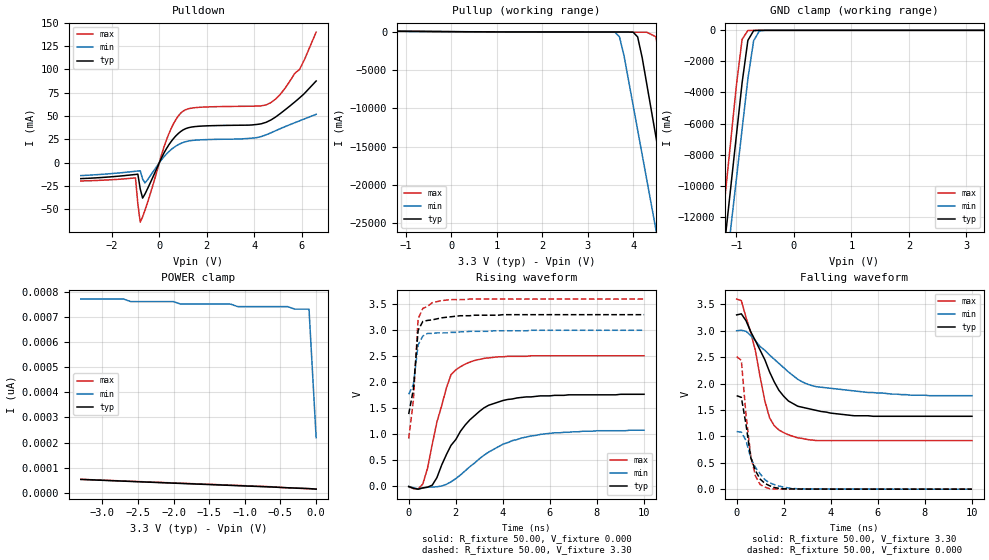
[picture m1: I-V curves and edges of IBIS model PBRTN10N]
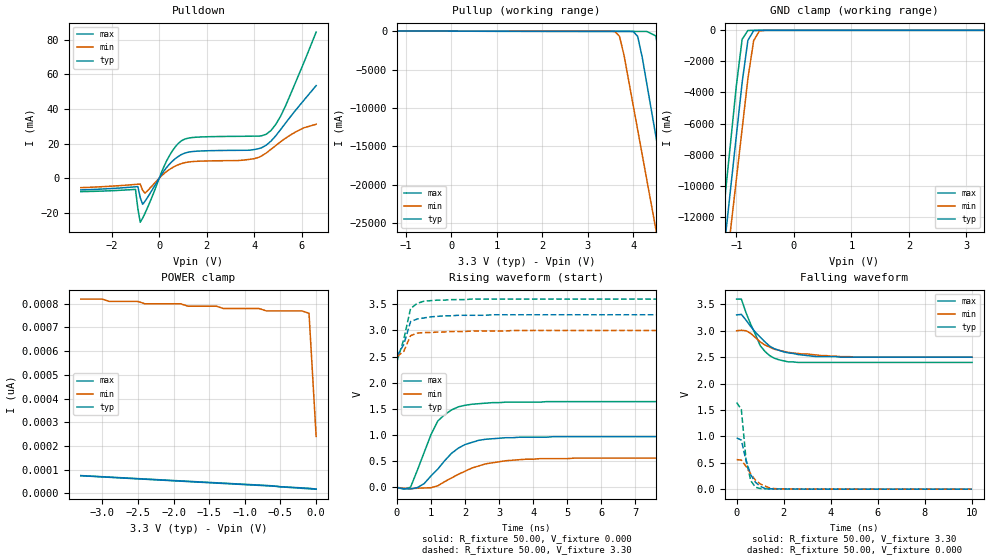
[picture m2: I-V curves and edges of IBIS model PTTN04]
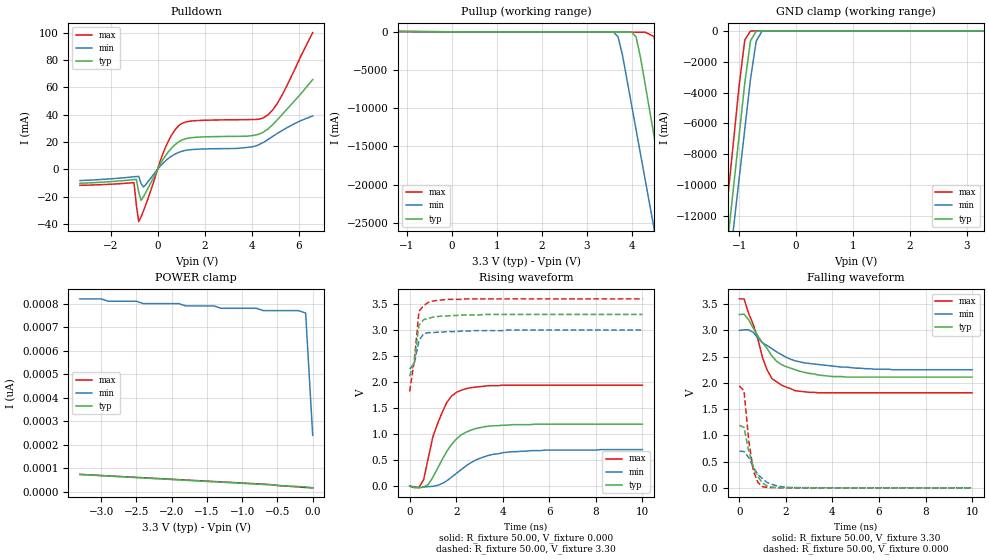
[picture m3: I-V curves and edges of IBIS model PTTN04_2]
| Integrated Devices Technolgy, Inc.
| IBIS MODEL OF 82v2048E
| PQFP_208
[Ibis Ver]   2.1
[File Name]   2048E_01.ibs
[File Rev]   2.0
[Date]   02/24/2002
[Source]   Integrated Devices Technolgy, Inc.
[Notes]   Spice type : spectre
[Disclaimer] Integrated Device Technology, Inc. ("IDT") hereby grants the
   user of this IBIS model a non-exclusive, nontransferable
   license to use this IBIS model under the following terms. The
   user is granted this license only to use the IBIS model and is
   not granted rights to sell, copy (except as needed to run the
   IBIS model), rent, lease or sub-license the IBIS model in
   whole or in part, or in modified form to anyone. The User may
   modify the IBIS model to suit its specific applications, but
   rights to derivative works and such modifications shall belong
   to IDT. This IBIS model is provided on an AS IS" basis and IDT
   makes absolutely no warranty with respect to the information
   contained herein. IDT DISCLAIMS AND CUSTOMER WAIVES ALL
   WARRANTIES, EXPRESS AND IMPLIED, INCLUDING WARRANTIES OF
   MERCHANTABILITY AND FITNESS FOR A PARTICULAR PURPOSE. THE
   ENTIRE RISK AS TO QUALITY AND PERFORMANCE IS WITH THE USER
   ACCORDINGLY, IN NO EVENT SHALL IDT BE LIABLE FOR ANY DIRECT OR
   INDIRECT DAMAGES, WHETHER IN CONTRACT OR TORT, INCLUDING ANY
   LOST PROFITS OR OTHER INCIDENTAL, CONSEQUENTIAL, EXEMPLARY, OR
   PUNITIVE DAMAGES ARISING OUT OF THE USE OR APPLICATION OF THE
   IBIS model. Further, IDT reserves the right to make changes
   without notice to any product herein to improve reliability,
   function, or design. IDT does not convey any license under
   patent rights or any other intellectual property rights,
   including those of third parties. IDT is not obligated to
   provide maintenance or support for the licensed IBIS model.
[Copyright]   Copyright 2002, Integrated Devices Technolgy, Inc. all rights
   reserved
|   Component 2048E_01 (PQFP_208)
[Component]   2048E_01
[Manufacturer]   Integrated Devices Technolgy, Inc.
[Package]
| variable   typ   min   max
R_pkg   178.7m   171.0m   186.4m
L_pkg   12.38nH   10.14nH   14.62nH
C_pkg   1.736pF   1.663pF   1.809pF
|   Pin List ( PQFP_208 )
[PIN]   signal_name   Model_name   R_pin   L_pin   C_pin
   1   LOS1   POTN04
   2   NC   NC
   3   LOS2   POTN04
   4   LOS3   POTN04
   5   LOS4   POTN04
   6   LOS5   POTN04
   7   LOS6   POTN04
   8   LOS7   POTN04
   9   LOS8   POTN04
   10   THZ   PITSN
   11   SCLKE   PITSN
   12   INT/MOT   PITSN
   13   IC   PITSN
   14   P/S   PITSN
   15   VDDD   POWER
   16   NC   NC
   17   MCLK   PITSN
   18   NC   NC
   19   GNDD   GND
   20   GNDIO   GND
   21   NC   NC
   22   VDDIO   POWER
   23   NC   NC
   24   D7   PBRTN10N
   25   D6   PBRTN10N
   26   D5   PBRTN10N
   27   D4   PBRTN10N
   28   D3   PBRTN10N
   29   D2   PBRTN10N
   30   D1   PBRTN10N
   31   D0   PBRTN10N
   32   NC   NC
   33   VDDIO   POWER
   34   TESTAPLL   POTN04
   35   GNDIO   GND
   36   NC   NC
   37   A7   PITSN
   38   A6   PITSN
   39   A5   PITSN
   40   A4   PITSN
   41   A3   PITSN
   42   A2   PITSN
   43   A1   PITSN
   44   A0   PITSN
   45   CS   PITSN
   46   SCLK   PITSN
   47   DS/RD   PITSN
   48   SDI/RW/WR   PITSN
   49   SDO   PTTN04_2
   50   INT   POTN04
   51   RST   PITSU
   52   NC   NC
   53   GPIO1   PBRTN10N
   54   GPIO0   PBRTN10N
   55   TESTSE   PITSN
   56   MCLKS   PITSN
   57   GNDA   GND
   58   TESTV   PAO
   59   REF   PAO
   60   VDDA   POWER
   61   VDDT   POWER
   62   VDDT   POWER
   63   TRING5   DRIVER
   64   TTIP5   DRIVER
   65   GNDT5   GND
   66   GNDT13   GND
   67   GNDR5   GND
   68   RRING5   PAI
   69   RTIP5   PAI
   70   VDDR5   POWER
   71   VDDR6   POWER
   72   RTIP6   PAI
   73   RRING6   PAI
   74   GNDR6   GND
   75   GNDT6   GND
   76   GNDT14   GND
   77   TTIP6   DRIVER
   78   TRING6   DRIVER
   79   VDDT   POWER
   80   VDDT   POWER
   81   VDDT   POWER
   82   VDDT   POWER
   83   TRING7   DRIVER
   84   TTIP7   DRIVER
   85   GNDT7   GND
   86   GNDT15   GND
   87   GNDR7   GND
   88   RRING7   PAI
   89   RTIP7   PAI
   90   VDDR7   POWER
   91   VDDR8   POWER
   92   RTIP8   PAI
   93   RRING8   PAI
   94   GNDR8   GND
   95   GNDT8   GND
   96   GNDT16   GND
   97   TTIP8   DRIVER
   98   TRING8   DRIVER
   99   VDDT   POWER
   100   VDDT   POWER
   101   NC   NC
   102   NC   NC
   103   VDDIO   POWER
   104   GNDIO   GND
   105   CV8/RDN8   PTTN04
   106   RD8/RDP8   PTTN04
   107   RCLK8   PTTN04_2
   108   TDN8   PITSN
   109   TD8/TDP8   PITSN
   110   TCLK8   PITSN
   111   CV7/RDN7   PTTN04
   112   RD7/RDP7   PTTN04
   113   RCLK7   PTTN04_2
   114   TDN7   PITSN
   115   TD7/TDP7   PITSN
   116   TCLK7   PITSN
   117   CV6/RDN6   PTTN04
   118   RD6/RDP6   PTTN04
   119   RCLK6   PTTN04_2
   120   TDN6   PITSN
   121   TD6/TDP6   PITSN
   122   TCLK6   PITSN
   123   CV5/RDN5   PTTN04
   124   RD5/RDP5   PTTN04
   125   RCLK5   PTTN04_2
   126   TDN5   PITSN
   127   TD5/TDP5   PITSN
   128   VDDIO   POWER
   129   TCLK5   PITSN
   130   GNDIO   GND
   131   GNDD   GND
   132   CV4/RDN4   PTTN04
   133   VDDD   POWER
   134   RD4/RDP4   PTTN04
   135   RCLK4   PTTN04_2
   136   TDN4   PITSN
   137   TD4/TDP4   PITSN
   138   TCLK4   PITSN
   139   CV3/RDN3   PTTN04
   140   RD3/RDP3   PTTN04
   141   RCLK3   PTTN04_2
   142   TDN3   PITSN
   143   TD3/TDP3   PITSN
   144   TCLK3   PITSN
   145   CV2/RDN2   PTTN04
   146   RD2/RDP2   PTTN04
   147   RCLK2   PTTN04_2
   148   TDN2   PITSN
   149   TD2/TDP2   PITSN
   150   TCLK2   PITSN
   151   CV1/RDN1   PTTN04
   152   RD1/RDP1   PTTN04
   153   RCLK1   PTTN04_2
   154   TDN1   PITSN
   155   TD1/TDP1   PITSN
   156   TCLK1   PITSN
   157   GNDIO   GND
   158   VDDIO   POWER
   159   NC   NC
   160   NC   NC
   161   VDDT   POWER
   162   VDDT   POWER
   163   TRING1   DRIVER
   164   TTIP1   DRIVER
   165   GNDT1   GND
   166   GNDT9   GND
   167   GNDR1   GND
   168   RRING1   PAI
   169   RTIP1   PAI
   170   VDDR1   POWER
   171   VDDR2   POWER
   172   RTIP2   PAI
   173   RRING2   PAI
   174   GNDR2   GND
   175   GNDT2   GND
   176   GNDT10   GND
   177   TTIP2   DRIVER
   178   TRING2   DRIVER
   179   VDDT   POWER
   180   VDDT   POWER
   181   VDDT   POWER
   182   VDDT   POWER
   183   TRING3   DRIVER
   184   TTIP3   DRIVER
   185   GNDT3   GND
   186   GNDT11   GND
   187   GNDR3   GND
   188   RRING3   PAI
   189   RTIP3   PAI
   190   VDDR3   POWER
   191   VDDR4   POWER
   192   RTIP4   PAI
   193   RRING4   PAI
   194   GNDR4   GND
   195   GNDT4   GND
   196   GNDT12   GND
   197   TTIP4   DRIVER
   198   TRING4   DRIVER
   199   VDDT   POWER
   200   VDDT   POWER
   201   VDDA   POWER
   202   NC   NC
   203   GNDA   GND
   204   TRST   PITSU
   205   TMS   PITSU
   206   TDI   PITSU
   207   TDO   PTTN04
   208   TCK   PITSN
| Models and submodels in the file (9): PBRTN10N (I/O), PTTN04 (3-state), PTTN04_2 (3-state), POTN04 (Output), PITSN (Input), PAI (Input), PITSU (Input), PAO (Input), DRIVER (3-state)
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|   Model PBRTN10N
[Model]   PBRTN10N
Model_type   I/O
Polarity   Non-Inverting
Enable   Active-Low
Vinl =   0.74V
Vinh =   2.10V
C_comp   3.50pF   4.00pF   3.20pF
[Temperature Range]   25.00   85.00   -40.00
[Voltage Range]   3.30V   3.00V   3.60V
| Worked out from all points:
|   slope of the pulldown table from 0 to 0.495 V, typ, clamps not added: 21.9 ohm
|   slope of the pullup table from 0 to 0.495 V, typ, clamps not added: 29.2 ohm
|   GND clamp passes 1 mA (typ) near -0.60 V on its own axis
|   rising waveform, R_fixture 50.00, V_fixture 0.000: 20-80 % time 1.59ns typ, 2.13ns min, 825ps max; typ from -0.002 V to 1.77 V
|   rising waveform, R_fixture 50.00, V_fixture 3.30: 20-80 % time 226ps typ, 225ps min, 235ps max; typ from 1.39 V to 3.3 V
|   falling waveform, R_fixture 50.00, V_fixture 3.30: 20-80 % time 1.32ns typ, 1.97ns min, 801ps max; typ from 3.3 V to 1.38 V
|   falling waveform, R_fixture 50.00, V_fixture 0.000: 20-80 % time 472ps typ, 702ps min, 384ps max; typ from 1.77 V to 0 V
[Pulldown]
| voltage   I(typ)   I(min)   I(max)
-3.3V     -16.95mA   -13.71mA   -19.45mA
-1V       -12.5mA    -9.06mA    -16.2mA
-900mV    -12.2mA    -8.75mA    -44.01mA
-800mV    -27.97mA   -8.57mA    -63.62mA
-700mV    -37.8mA    -17.39mA   -57.93mA
-600mV    -33.43mA   -21.55mA   -50.78mA
300mV     15.03mA    9.35mA     24.27mA
900mV     33.46mA    20.65mA    53.15mA
1.5V      38.77mA    24.19mA    59.03mA
4.7V      45.89mA    32.14mA    64.49mA
5.9V      69.46mA    44.93mA    100mA
6.6V      87.62mA    51.95mA    140mA
[Pullup]
| voltage   I(typ)   I(min)   I(max)
-3.3V     120mA      79.67mA    180mA
3.6V      -41.5mA    -64.51mA   -72.86mA
3.7V      -41.65mA   -690mA     -73.1mA
3.8V      -41.8mA    -3.15A     -73.33mA
4.1V      -690mA     -12.84A    -73.96mA
4.3V      -6.82A     -19.3A     -75.1mA
4.5V      -13.65A    -25.76A    -660mA
4.7V      -20.47A    -32.21A    -7.27A
4.9V      -27.29A    -38.67A    -14.54A
5.1V      -34.12A    -45.13A    -21.81A
5.3V      -40.94A    -51.59A    -29.07A
6.6V      -85.3A     -93.57A    -76.32A
[GND_clamp]
| voltage   I(typ)   I(min)   I(max)
-3.3V     -85.25A    -83.86A    -87.14A
-1.3V     -17.02A    -19.27A    -14.46A
-1.2V     -13.61A    -16.05A    -10.83A
-1.1V     -10.19A    -12.82A    -7.2A
-1V       -6.78A     -9.59A     -3.56A
-900mV    -3.37A     -6.36A     -580mA
-800mV    -650mA     -3.13A     -10.84mA
-700mV    -23.03mA   -670mA     -750uA
-600mV    -570uA     -40.72mA   -46.43uA
-400mV    -420nA     -76.92uA   -33.22nA
3.3V      15.23pA    730pA      12.85pA
[POWER_clamp]
| voltage   I(typ)   I(min)   I(max)
-3.3V     53.95pA    770pA      54.34pA
-2.7V     47.02pA    770pA      47.72pA
-2.6V     45.88pA    760pA      46.62pA
-2V       39.11pA    760pA      40.01pA
-1.9V     37.99pA    750pA      38.91pA
-1.2V     30.19pA    750pA      31.21pA
-1.1V     29.08pA    740pA      30.11pA
-400mV    20.85pA    740pA      20.54pA
-300mV    19.76pA    730pA      19.3pA
-100mV    17.59pA    730pA      17.04pA
0V        15.23pA    220pA      15.99pA
[Ramp]
| variable   typ   min   max
dV/dt_r   1.06/1.42n   0.65/2.13n   1.51/0.80n
dV/dt_f   1.15/1.32n   0.74/1.94n   1.61/0.81n
R_load = 50.00
[Rising Waveform]
R_fixture = 50.00
V_fixture = 0.000
V_fixture_min = 0.000
V_fixture_max = 0.000
| time   V(typ)   V(min)   V(max)
0s        -2.35mV    -1.01mV    -3.76mV
600ps     -28.68mV   -31.05mV   45.89mV
1ns       23.7mV     -11.09mV   810mV
1.6ns     610mV      39.29mV    1.89V
1.8ns     790mV      88.39mV    2.15V
2.2ns     1.06V      220mV      2.3V
3.2ns     1.51V      600mV      2.46V
4.2ns     1.67V      840mV      2.5V
6.2ns     1.75V      1.03V      2.51V
10ns      1.77V      1.08V      2.51V
[Rising Waveform]
R_fixture = 50.00
V_fixture = 3.30
V_fixture_min = 3.00
V_fixture_max = 3.60
| time   V(typ)   V(min)   V(max)
0s        1.39V      1.77V      920mV
200ps     1.87V      1.96V      1.66V
400ps     3V         2.72V      3.22V
600ps     3.17V      2.89V      3.42V
800ps     3.19V      2.94V      3.46V
1ns       3.2V       2.94V      3.53V
1.8ns     3.26V      2.96V      3.59V
2.8ns     3.29V      2.98V      3.6V
5.2ns     3.3V       3V         3.6V
10ns      3.3V       3V         3.6V
[Falling Waveform]
R_fixture = 50.00
V_fixture = 3.30
V_fixture_min = 3.00
V_fixture_max = 3.60
| time   V(typ)   V(min)   V(max)
0s        3.3V       3V         3.6V
200ps     3.32V      3.01V      3.57V
600ps     2.98V      2.91V      2.97V
800ps     2.81V      2.81V      2.62V
1.2ns     2.45V      2.63V      1.67V
1.4ns     2.22V      2.54V      1.35V
1.8ns     1.87V      2.38V      1.12V
2.6ns     1.57V      2.08V      970mV
3.4ns     1.49V      1.94V      920mV
10ns      1.38V      1.77V      920mV
[Falling Waveform]
R_fixture = 50.00
V_fixture = 0.000
V_fixture_min = 0.000
V_fixture_max = 0.000
| time   V(typ)   V(min)   V(max)
0s        1.77V      1.09V      2.51V
200ps     1.74V      1.08V      2.44V
400ps     1.22V      920mV      1.4V
600ps     600mV      590mV      630mV
800ps     350mV      410mV      250mV
1ns       190mV      290mV      86.54mV
1.4ns     65.04mV    120mV      8.44mV
1.8ns     15.51mV    59.38mV    3.46mV
2.4ns     4.08mV     13.27mV    1.63mV
10ns      1.37uV     -16.49uV   -7.85uV
|   Model PTTN04
[Model]   PTTN04
Model_type   3-state
Polarity   Non-Inverting
Enable   Active-Low
C_comp   3.50pF   4.00pF   3.50pF
[Temperature Range]   25.00   85.00   -40.00
[Voltage Range]   3.30V   3.00V   3.60V
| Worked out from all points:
|   slope of the pulldown table from 0 to 0.495 V, typ, clamps not added: 54.8 ohm
|   slope of the pullup table from 0 to 0.495 V, typ, clamps not added: 58.3 ohm
|   GND clamp passes 1 mA (typ) near -0.60 V on its own axis
|   rising waveform, R_fixture 50.00, V_fixture 0.000: 20-80 % time 911ps typ, 1.18ns min, 672ps max; typ from -0.001 V to 0.97 V
|   rising waveform, R_fixture 50.00, V_fixture 3.30: 20-80 % time 244ps typ, 200ps min, 267ps max; typ from 2.51 V to 3.3 V
|   falling waveform, R_fixture 50.00, V_fixture 3.30: 20-80 % time 1.1ns typ, 1.37ns min, 761ps max; typ from 3.3 V to 2.5 V
|   falling waveform, R_fixture 50.00, V_fixture 0.000: 20-80 % time 430ps typ, 596ps min, 274ps max; typ from 0.97 V to 0 V
[Pulldown]
| voltage   I(typ)   I(min)   I(max)
-3.3V     -6.78mA    -5.48mA    -7.78mA
-1V       -5mA       -3.62mA    -6.48mA
-900mV    -4.88mA    -3.5mA     -17.6mA
-800mV    -11.19mA   -3.43mA    -25.45mA
-700mV    -15.12mA   -6.95mA    -23.17mA
-600mV    -13.37mA   -8.62mA    -20.31mA
300mV     6.01mA     3.74mA     9.71mA
900mV     13.39mA    8.26mA     21.26mA
3.9V      16.33mA    11.07mA    24.26mA
4.7V      21.41mA    16.66mA    27.53mA
5.3V      31.61mA    22.97mA    41.38mA
6.6V      53.5mA     31.16mA    84.43mA
[Pullup]
| voltage   I(typ)   I(min)   I(max)
-3.3V     75.1mA     45.9mA     110mA
3.6V      -20.75mA   -52.61mA   -36.43mA
3.7V      -20.82mA   -680mA     -36.55mA
3.8V      -20.91mA   -3.14A     -36.66mA
4.1V      -670mA     -12.83A    -36.98mA
4.3V      -6.8A      -19.29A    -37.92mA
4.5V      -13.63A    -25.74A    -620mA
4.7V      -20.45A    -32.2A     -7.23A
4.9V      -27.27A    -38.66A    -14.5A
5.1V      -34.1A     -45.12A    -21.77A
5.3V      -40.92A    -51.58A    -29.04A
6.6V      -85.27A    -93.56A    -76.28A
[GND_clamp]
| voltage   I(typ)   I(min)   I(max)
-3.3V     -85.25A    -83.86A    -87.14A
-1.3V     -17.02A    -19.27A    -14.46A
-1.2V     -13.61A    -16.05A    -10.83A
-1.1V     -10.19A    -12.82A    -7.2A
-1V       -6.78A     -9.59A     -3.56A
-900mV    -3.37A     -6.36A     -580mA
-800mV    -650mA     -3.13A     -10.84mA
-700mV    -23.03mA   -670mA     -750uA
-600mV    -570uA     -40.72mA   -46.43uA
-400mV    -420nA     -76.92uA   -33.22nA
3.3V      17.37pA    770pA      12.87pA
[POWER_clamp]
| voltage   I(typ)   I(min)   I(max)
-3.3V     73.8pA     820pA      74.49pA
-2.5V     60.59pA    810pA      61.66pA
-2.4V     58.95pA    800pA      60.06pA
-1.9V     50.83pA    800pA      52.05pA
-1.8V     49.21pA    790pA      50.45pA
-1.4V     42.75pA    790pA      44.05pA
-1.3V     41.14pA    780pA      42.44pA
-800mV    33.09pA    780pA      34.44pA
-700mV    31.48pA    770pA      32.83pA
-200mV    22.54pA    770pA      20.69pA
-100mV    20.96pA    760pA      18.49pA
0V        17.27pA    240pA      17.07pA
[Ramp]
| variable   typ   min   max
dV/dt_r   0.58/0.86n   0.34/1.22n   0.98/0.61n
dV/dt_f   0.48/1.02n   0.30/1.52n   0.72/0.71n
R_load = 50.00
[Rising Waveform]
R_fixture = 50.00
V_fixture = 0.000
V_fixture_min = 0.000
V_fixture_max = 0.000
| time   V(typ)   V(min)   V(max)
0s        -1.28mV    -400uV     -2.34mV
200ps     -25mV      -16.44mV   -33.49mV
400ps     -28.55mV   -25.32mV   4.49mV
800ps     73.89mV    -10.55mV   670mV
1ns       220mV      -5.62mV    1.01V
1.2ns     350mV      31.07mV    1.27V
1.8ns     750mV      250mV      1.54V
2.4ns     900mV      410mV      1.6V
3.8ns     960mV      540mV      1.63V
10ns      970mV      560mV      1.64V
[Rising Waveform]
R_fixture = 50.00
V_fixture = 3.30
V_fixture_min = 3.00
V_fixture_max = 3.60
| time   V(typ)   V(min)   V(max)
0s        2.51V      2.5V       2.41V
200ps     2.73V      2.6V       2.83V
400ps     3.17V      2.9V       3.42V
600ps     3.22V      2.95V      3.52V
800ps     3.24V      2.96V      3.56V
1.4ns     3.28V      2.97V      3.58V
2.2ns     3.29V      2.99V      3.6V
2.8ns     3.3V       2.99V      3.6V
3.4ns     3.3V       3V         3.6V
10ns      3.3V       3V         3.6V
[Falling Waveform]
R_fixture = 50.00
V_fixture = 3.30
V_fixture_min = 3.00
V_fixture_max = 3.60
| time   V(typ)   V(min)   V(max)
0s        3.3V       3V         3.6V
200ps     3.31V      3.01V      3.6V
600ps     3.08V      2.95V      3.12V
1ns       2.88V      2.79V      2.72V
1.4ns     2.71V      2.69V      2.53V
1.8ns     2.63V      2.63V      2.45V
2.2ns     2.58V      2.59V      2.41V
3.4ns     2.51V      2.54V      2.4V
5ns       2.5V       2.5V       2.4V
10ns      2.5V       2.5V       2.4V
[Falling Waveform]
R_fixture = 50.00
V_fixture = 0.000
V_fixture_min = 0.000
V_fixture_max = 0.000
| time   V(typ)   V(min)   V(max)
0s        970mV      560mV      1.64V
200ps     930mV      550mV      1.51V
400ps     540mV      430mV      560mV
600ps     270mV      290mV      160mV
800ps     130mV      170mV      38.48mV
1ns       56mV       100mV      11.04mV
1.2ns     12.7mV     59.65mV    7.28mV
1.4ns     7.26mV     23.89mV    4.27mV
1.8ns     4.54mV     6.11mV     1.29mV
10ns      1.93uV     9.71uV     820nV
|   Model PTTN04_2
[Model]   PTTN04_2
Model_type   3-state
Polarity   Non-Inverting
Enable   Active-Low
C_comp   3.50pF   4.00pF   3.50pF
[Temperature Range]   25.00   85.00   -40.00
[Voltage Range]   3.30V   3.00V   3.60V
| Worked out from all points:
|   slope of the pulldown table from 0 to 0.495 V, typ, clamps not added: 36.6 ohm
|   slope of the pullup table from 0 to 0.495 V, typ, clamps not added: 46.6 ohm
|   GND clamp passes 1 mA (typ) near -0.60 V on its own axis
|   rising waveform, R_fixture 50.00, V_fixture 0.000: 20-80 % time 1.05ns typ, 1.49ns min, 812ps max; typ from -0.002 V to 1.19 V
|   rising waveform, R_fixture 50.00, V_fixture 3.30: 20-80 % time 233ps typ, 259ps min, 255ps max; typ from 2.11 V to 3.3 V
|   falling waveform, R_fixture 50.00, V_fixture 3.30: 20-80 % time 1.24ns typ, 1.8ns min, 816ps max; typ from 3.3 V to 2.11 V
|   falling waveform, R_fixture 50.00, V_fixture 0.000: 20-80 % time 481ps typ, 664ps min, 314ps max; typ from 1.19 V to 0 V
[Pulldown]
| voltage   I(typ)   I(min)   I(max)
-3.3V     -10.17mA   -8.22mA    -11.67mA
-1V       -7.5mA     -5.43mA    -9.72mA
-900mV    -7.32mA    -5.25mA    -26.41mA
-800mV    -16.78mA   -5.14mA    -38.17mA
-700mV    -22.68mA   -10.43mA   -34.76mA
-600mV    -20.06mA   -12.93mA   -30.47mA
300mV     9.02mA     5.61mA     14.56mA
800mV     18.81mA    11.62mA    30.08mA
1.3V      22.8mA     14.17mA    34.98mA
4.7V      29.57mA    21.83mA    39.85mA
5.3V      40.09mA    28.41mA    54.3mA
6.6V      65.68mA    39.04mA    100mA
[Pullup]
| voltage   I(typ)   I(min)   I(max)
-3.3V     86.33mA    53.19mA    130mA
3.6V      -25.94mA   -55.59mA   -45.54mA
3.7V      -26.03mA   -680mA     -45.69mA
3.8V      -26.13mA   -3.14A     -45.83mA
4.1V      -680mA     -12.83A    -46.23mA
4.3V      -6.81A     -19.29A    -47.22mA
4.5V      -13.63A    -25.75A    -630mA
4.7V      -20.46A    -32.21A    -7.24A
4.9V      -27.28A    -38.66A    -14.51A
5.1V      -34.1A     -45.12A    -21.78A
5.3V      -40.93A    -51.58A    -29.05A
6.6V      -85.28A    -93.56A    -76.29A
[GND_clamp]
| voltage   I(typ)   I(min)   I(max)
-3.3V     -85.25A    -83.86A    -87.14A
-1.3V     -17.02A    -19.27A    -14.46A
-1.2V     -13.61A    -16.05A    -10.83A
-1.1V     -10.19A    -12.82A    -7.2A
-1V       -6.78A     -9.59A     -3.56A
-900mV    -3.37A     -6.36A     -580mA
-800mV    -650mA     -3.13A     -10.84mA
-700mV    -23.03mA   -670mA     -750uA
-600mV    -570uA     -40.72mA   -46.43uA
-400mV    -420nA     -76.92uA   -33.22nA
3.3V      17.37pA    770pA      12.85pA
[POWER_clamp]
| voltage   I(typ)   I(min)   I(max)
-3.3V     73.8pA     820pA      74.44pA
-2.5V     60.58pA    810pA      61.62pA
-2.4V     58.95pA    800pA      60.02pA
-1.9V     50.82pA    800pA      52.01pA
-1.8V     49.21pA    790pA      50.41pA
-1.4V     42.75pA    790pA      44.01pA
-1.3V     41.13pA    780pA      42.41pA
-800mV    33.09pA    780pA      34.41pA
-700mV    31.48pA    770pA      32.8pA
-200mV    22.54pA    770pA      20.66pA
-100mV    20.96pA    760pA      18.46pA
0V        17.27pA    240pA      17.04pA
[Ramp]
| variable   typ   min   max
dV/dt_r   0.72/1.04n   0.42/1.49n   1.17/0.70n
dV/dt_f   0.71/1.19n   0.45/1.73n   1.07/0.81n
R_load = 50.00
[Rising Waveform]
R_fixture = 50.00
V_fixture = 0.000
V_fixture_min = 0.000
V_fixture_max = 0.000
| time   V(typ)   V(min)   V(max)
0s        -1.51mV    -530uV     -2.62mV
400ps     -35.79mV   -32.19mV   -25.03mV
600ps     -19.18mV   -19.59mV   120mV
1ns       170mV      -7.41mV    950mV
1.4ns     510mV      48.34mV    1.42V
1.8ns     800mV      170mV      1.73V
2.2ns     980mV      310mV      1.84V
3ns       1.12V      530mV      1.91V
4ns       1.17V      640mV      1.94V
10ns      1.19V      700mV      1.94V
[Rising Waveform]
R_fixture = 50.00
V_fixture = 3.30
V_fixture_min = 3.00
V_fixture_max = 3.60
| time   V(typ)   V(min)   V(max)
0s        2.11V      2.25V      1.82V
200ps     2.41V      2.36V      2.41V
400ps     3.09V      2.8V       3.36V
600ps     3.2V       2.93V      3.47V
800ps     3.22V      2.95V      3.53V
1ns       3.25V      2.95V      3.56V
1.6ns     3.27V      2.97V      3.59V
2.2ns     3.29V      2.98V      3.59V
3.2ns     3.3V       2.99V      3.6V
10ns      3.3V       3V         3.6V
[Falling Waveform]
R_fixture = 50.00
V_fixture = 3.30
V_fixture_min = 3.00
V_fixture_max = 3.60
| time   V(typ)   V(min)   V(max)
0s        3.3V       3V         3.6V
200ps     3.31V      3.01V      3.6V
600ps     3.04V      2.96V      3.11V
1ns       2.76V      2.76V      2.47V
1.2ns     2.65V      2.71V      2.24V
1.4ns     2.51V      2.65V      2.08V
2ns       2.31V      2.49V      1.92V
2.4ns     2.25V      2.42V      1.85V
4ns       2.12V      2.32V      1.81V
10ns      2.11V      2.25V      1.81V
[Falling Waveform]
R_fixture = 50.00
V_fixture = 0.000
V_fixture_min = 0.000
V_fixture_max = 0.000
| time   V(typ)   V(min)   V(max)
0s        1.19V      700mV      1.94V
200ps     1.15V      690mV      1.85V
400ps     710mV      580mV      910mV
600ps     400mV      390mV      320mV
800ps     210mV      250mV      99.86mV
1ns       88.8mV     170mV      21.99mV
1.2ns     33.22mV    99.38mV    7.33mV
1.4ns     12.02mV    66.22mV    5.32mV
2.2ns     3.35mV     5.86mV     780uV
10ns      -1.47uV    2.87uV     780nV
